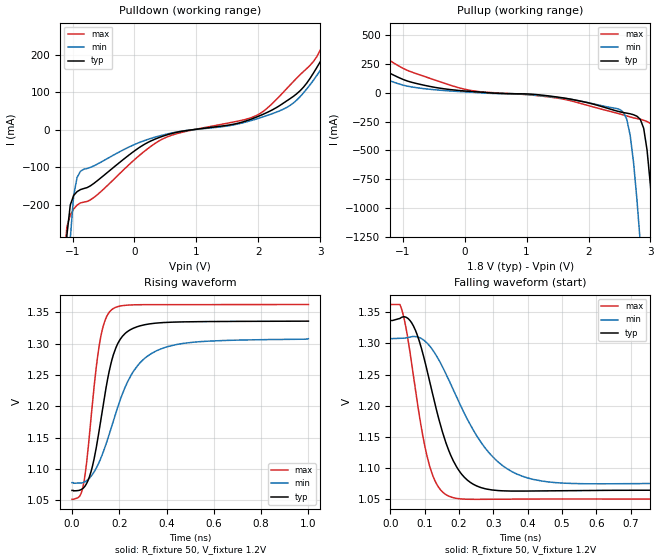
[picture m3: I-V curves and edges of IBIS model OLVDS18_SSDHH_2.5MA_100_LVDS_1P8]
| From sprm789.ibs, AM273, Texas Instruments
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|   Model Cell OLVDS18_SSDHH_2.5MA_100_LVDS_1P8
|OLVDS18_SSDHH_2.5MA_100_LVDS_1P8
[Model]   OLVDS18_SSDHH_2.5MA_100_LVDS_1P8
Model_type   Output
Polarity   Non-Inverting
Cref =  15.0001pF
Rref =  101.0000M
Vref =  0V
Vmeas =  1.08
C_comp   1.5p   1.5p   1.5p
[Temperature Range]   25   125   -40
[Voltage Range]   1.8   1.62   1.98
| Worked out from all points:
|   slope of the pulldown table from 0 to 0.27 V, typ, clamps not added: 10 ohm
|   slope of the pullup table from 0 to 0.27 V, typ, clamps not added: 26.7 ohm
|   rising waveform, R_fixture 50, V_fixture 1.2V: 20-80 % time 79.2ps typ, 142ps min, 53.7ps max; typ from 1.07 V to 1.34 V
|   falling waveform, R_fixture 50, V_fixture 1.2V: 20-80 % time 81.7ps typ, 137ps min, 56.5ps max; typ from 1.34 V to 1.06 V
| Nom Voltages:
|   BIAS1=1.2, BIAS2=1.2, VDD=1.1, VDDS=1.8, BUS_BIAS3=0, BUS_VSSS=0,
|   ESD_BIASFET=0, VSS=0
| Min Voltages:
|   BIAS1=1.2, BIAS2=1.2, VDD=0.99, VDDS=1.62, BUS_BIAS3=0, BUS_VSSS=0,
|   ESD_BIASFET=0, VSS=0
| Max Voltages:
|   BIAS1=1.2, BIAS2=1.2, VDD=1.21, VDDS=1.98, BUS_BIAS3=0, BUS_VSSS=0,
|   ESD_BIASFET=0, VSS=0
[Pulldown]
|   voltage   I(typ)   I(min)   I(max)
-1.8V     -6.003A    -6.315A    -5.869A
-1.091V   -280.6mA   -503.9mA   -258.7mA
-1.036V   -200.4mA   -290.5mA   -227mA
-981.8mV  -175mA     -174.8mA   -211.2mA
-872.7mV  -159.5mA   -110.7mA   -195mA
-109.1mV  -70.02mA   -47.71mA   -96.31mA
545.5mV   -12.59mA   -10.66mA   -17.98mA
1.964V    33.25mA    28.37mA    37.5mA
2.509V    82.38mA    64.42mA    118.5mA
3.164V    227.1mA    199.7mA    283.1mA
3.382V    294.4mA    298.5mA    391.7mA
3.6V      374.2mA    801.1mA    517.9mA
[Pullup]
|   voltage   I(typ)   I(min)   I(max)
-1.8V     324mA      320.6mA    560.6mA
-1.2V     167.4mA    102.1mA    276mA
-218.2mV  26.86mA    14.81mA    63.47mA
2.509V    -165.7mA   -146.4mA   -184.3mA
2.673V    -182.5mA   -368.3mA   -209.9mA
2.782V    -203.4mA   -924.6mA   -223.9mA
2.836V    -230.4mA   -1.302A    -229.5mA
2.945V    -496.7mA   -2.158A    -250mA
3.055V    -1.187A    -3.089A    -291.3mA
3.164V    -2.07A     -4.052A    -542.9mA
3.273V    -3.029A    -5.017A    -1.279A
3.6V      -6.007A    -7.911A    -4.201A
[Ramp]
| variable   typ   min   max
dV/dt_f 0.16132644/98.040276p 0.13431336/0.15353422n  0.1912465/71.946276p
dV/dt_r 0.20822262/0.10526012n 0.16533065/0.16637923n 0.24446713/73.403736p
R_load = 50
[Rising Waveform]
R_fixture = 50
V_fixture = 1.2V
V_fixture_min = 1.2V
V_fixture_max = 1.2V
|   time   V(typ)   V(min)   V(max)
0s        1.066V     1.078V     1.052V
45.14ps   1.069V     1.078V     1.069V
78.67ps   1.093V     1.088V     1.173V
101.7ps   1.132V     1.101V     1.26V
121.5ps   1.177V     1.117V     1.311V
167.9ps   1.273V     1.168V     1.354V
201.8ps   1.306V     1.208V     1.36V
259.9ps   1.325V     1.256V     1.362V
364.3ps   1.333V     1.29V      1.363V
1ns       1.336V     1.308V     1.363V
[Falling Waveform]
R_fixture = 50
V_fixture = 1.2V
V_fixture_min = 1.2V
V_fixture_max = 1.2V
|   time   V(typ)   V(min)   V(max)
0s        1.336V     1.307V     1.362V
33.51ps   1.342V     1.308V     1.353V
70.33ps   1.324V     1.311V     1.236V
114.8ps   1.238V     1.296V     1.103V
163.5ps   1.138V     1.249V     1.057V
199.8ps   1.096V     1.206V     1.051V
240.6ps   1.075V     1.162V     1.05V
302.6ps   1.065V     1.116V     1.051V
380.9ps   1.063V     1.088V     1.051V
1ns       1.065V     1.077V     1.051V
